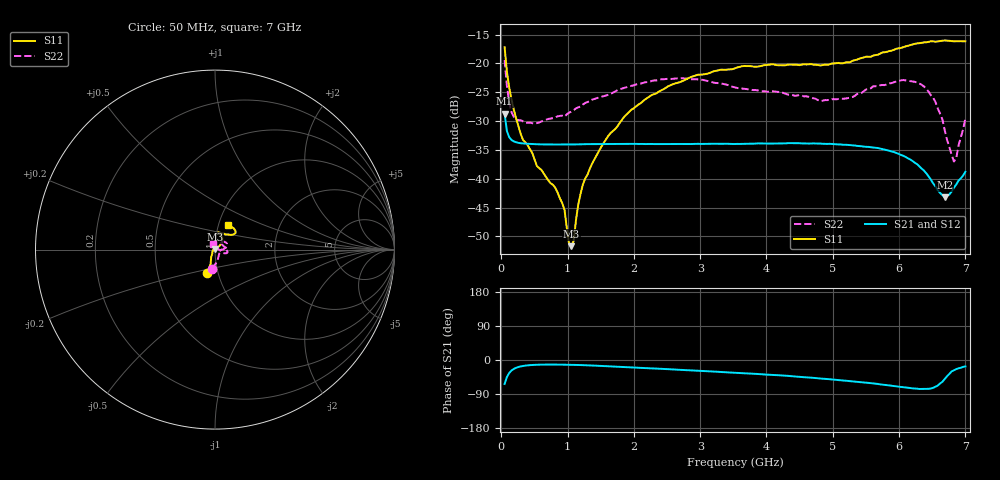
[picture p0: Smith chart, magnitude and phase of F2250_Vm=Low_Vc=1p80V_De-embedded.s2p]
! Integrated Device Technology
! Corporate Headquarters
! 6024 Silver Creek Valley Road
! San Jose, CA 95138  USA
! Phone:  1-408-284-8200
! Toll Free:  1-800-223-1366
! Webpage:  http://www.idt.com/
! Timing and RF Division
! 515 Groton Road, Suite 102
! Westford, MA 01886-6024
! Device:  F2250
! Description: Voltage Variable RF Attenuator
! Frequency:  50.0 -  6000.00 MHz
! Package:  3x3 mm Thin QFN Plastic Package: 16 pin
! Ports:  2 RF, 3 DC
!  Pin  1  = GND
!  Pin  2  = NC
!  Pin  3  = RF1  = Port 1
!  Pin  4  = NC
!  Pin  5  = GND
!  Pin  6  = GND
!  Pin  7  = GND
!  Pin  8  = GND
!  Pin  9  = NC
!  Pin 10  = RF2  = Port 2
!  Pin 11  = NC
!  Pin 12  = GND
!  Pin 13  = GND
!  Pin 14  = VCNTRL
!  Pin 15  = VDD
!  Pin 16  = VMODE
! Vcntrl:  1.800 Volts
! Vmode:  +0.000 Volts
! Vdd:  +3.30  Volts
! Current:  1.186 mA
! Data:  The device was measured on a the F2250 evaluation board which has
!  individual transmission lines to the RF pins.  Data was collected
!  using a calibrated network analyzer.  The evaluation board was
!  de-embedded using a TRL calibration technique.
!  The reference plane is the edge of the package pin.
! Misc:  SN 10
!  Action Tracker AT0258
! Date Measured:  2014-11-26
! Date:  2015-10-15  MJV
! Note:
!  Integrated Device Technology supplies this data as a sample of measured
!  data at the package pin for this product.  Your particular data for this
!  product may vary.
!  Data was taken at 25 degrees C.
!  Integrated Device Technology reserves the right to change this data at anytime.
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# GHz S dB R 50
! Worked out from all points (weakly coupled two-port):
!   201 points, 50 MHz to 7 GHz, reference 50 ohm
!   highest |S21| = -28.72 dB at 50 MHz (marker M1); lowest = -43.2 dB at 6.687 GHz (marker M2)
!   lowest |S11| = -51.7 dB at 1.058 GHz (marker M3), VSWR 1.01, Z = 49.9 + j0.233 ohm
!   |S11| at or under -10 dB: start of sweep to end of sweep
!   |S22| runs from -37.0 to -19.4 dB; largest |S21 - S12| = 5.8e-05
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0.05  -17.17 -108.4  -28.72 -63.3  -28.72 -63.3  -19.41 -97.6
0.1195  -24.20 -111.3  -32.80 -34.2  -32.80 -34.2  -26.77 -66.0
0.22375  -29.54 -121.5  -33.67 -20.6  -33.67 -20.6  -29.74 -41.5
0.5365  -37.79 -154.3  -34.01 -12.5  -34.01 -12.5  -30.34 -8.7
0.91875  -44.21 158.1  -34.07 -12.3  -34.07 -12.3  -29.03 -3.0
0.9535  -45.38 170.0  -34.07 -12.4  -34.06 -12.4  -29.22 -1.4
1.023  -51.37 142.1  -34.06 -12.6  -34.06 -12.6  -28.53 0.6
1.05775  -51.70 116.2  -34.06 -12.7  -34.06 -12.7  -28.35 1.5
1.0925  -50.75 83.1  -34.05 -12.9  -34.05 -12.8  -28.10 1.1
1.162  -44.41 52.7  -34.04 -13.2  -34.03 -13.2  -27.60 0.6
1.2315  -40.96 41.4  -34.01 -13.6  -34.01 -13.5  -27.12 0.4
1.6485  -32.06 40.9  -33.97 -16.7  -33.96 -16.6  -25.27 8.0
2.37825  -24.87 46.9  -33.96 -23.1  -33.97 -23.1  -22.84 18.5
3.525  -20.83 72.3  -33.97 -33.5  -33.97 -33.5  -24.16 45.8
4.7065  -20.20 72.2  -33.86 -47.2  -33.87 -47.2  -26.03 52.4
5.22775  -19.81 56.2  -34.12 -55.2  -34.12 -55.2  -26.01 26.9
5.85325  -17.84 40.3  -35.15 -67.2  -35.14 -67.2  -23.45 -4.6
6.3745  -16.35 41.3  -38.57 -76.5  -38.59 -76.5  -23.98 -18.9
6.54825  -16.20 45.0  -41.34 -70.5  -41.36 -70.4  -26.66 -21.1
6.68725  -16.00 48.7  -43.23 -50.1  -43.25 -49.7  -31.51 -6.2
6.82625  -16.15 53.5  -41.57 -27.1  -41.53 -27.1  -37.01 48.1
7  -16.14 63.2  -38.78 -17.1  -38.75 -17.2  -29.51 109.8
